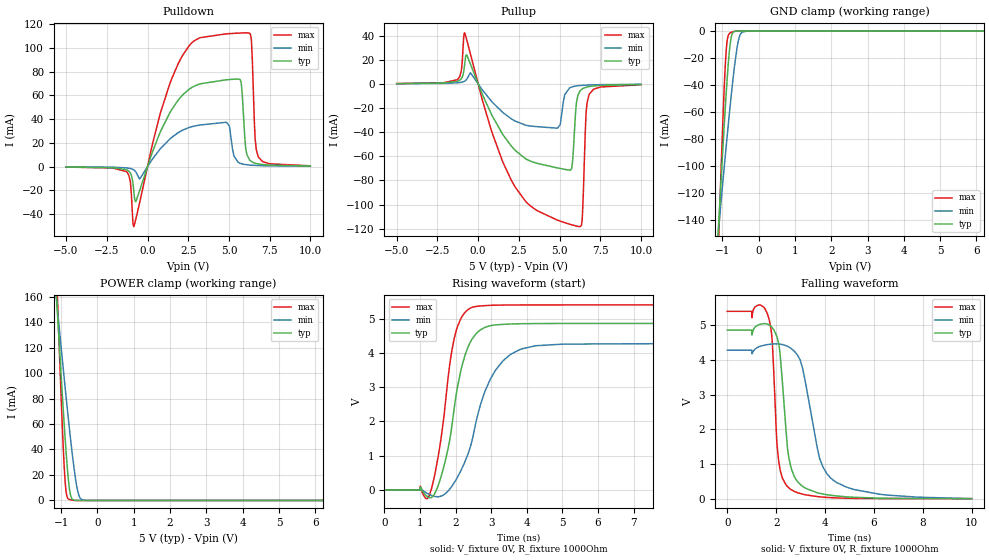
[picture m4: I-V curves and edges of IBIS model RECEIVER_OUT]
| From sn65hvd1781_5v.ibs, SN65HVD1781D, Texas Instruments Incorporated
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|   RECEIVER_OUT Model
[Model]   RECEIVER_OUT
Model_type   Output
| Signals   R
Polarity   Non-Inverting
Enable   Active-High
Vmeas = 2.5
Vref = 2.5
Cref = 15pF
Rref = 1000
| variable   typ   min   max
C_comp   0.74pF   0.68pF   0.82pF
|   typ   min   max
[Voltage Range]   5   4.5   5.5
[Temperature Range]   25   150   -40
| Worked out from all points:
|   slope of the pulldown table from 0 to 0.75 V, typ, clamps not added: 26.6 ohm
|   slope of the pullup table from 0 to 0.75 V, typ, clamps not added: 32.1 ohm
|   GND clamp passes 1 mA (typ) near -0.70 V on its own axis
|   POWER clamp passes 1 mA (typ) near -0.69 V on its own axis
|   falling waveform, V_fixture 0V, R_fixture 1000Ohm: 20-80 % time 387ps typ, 786ps min, 249ps max; typ from 4.86 V to -0.001 V
|   rising waveform, V_fixture 0V, R_fixture 1000Ohm: 20-80 % time 514ps typ, 806ps min, 415ps max; typ from -0.001 V to 4.86 V
[Pulldown]
| Non-monotonic behavior is expected as a consequence of circuit design
|   Voltage   I(typ)   I(min)   I(max)
-5V       -292.3uA   -182.5uA   -355.9uA
-1.295V   -2.615mA   -1.069mA   -4.183mA
-845mV    -20.19mA   -2.707mA   -50.61mA
812.5mV   30.03mA    15.41mA    46.12mA
2.163V    60.52mA    30.8mA     93.99mA
4.855V    73.27mA    37.4mA     112.1mA
5.695V    73.32mA    2.76mA     112.7mA
6.055V    13.33mA    1.64mA     112.9mA
6.362V    4.439mA    1.213mA    108.7mA
6.603V    2.888mA    1.007mA    24.61mA
6.798V    2.245mA    884.5uA    8.31mA
9.992V    476.5uA    293.2uA    664.2uA
[GND Clamp]
| High Current due to TISpice simulations which do not match silicon
| High operating voltage drives high currents.
| Non-monotonic behavior is expected near 0V with small currents.
|   Voltage   I(typ)   I(min)   I(max)
-5V       -2.27A     -1.411A    -3.663A
-1.107V   -146mA     -147.8mA   -160.6mA
-1.093V   -138.6mA   -143.4mA   -148.6mA
-987.5mV  -88.11mA   -112.4mA   -68.55mA
-905mV    -51.15mA   -88.69mA   -19.27mA
-860mV    -33.03mA   -76.05mA   -5.989mA
-807.5mV  -15.47mA   -61.68mA   -1.94mA
-725mV    -1.911mA   -40.27mA   -630.7uA
-597.5mV  -18.86uA   -12.9mA    -19.83uA
-537.5mV  18.77uA    -4.964mA   15.69uA
-297.5mV  25.6uA     9.488uA    22.75uA
10V       0A         0A         0A
[Pullup]
| Non-monotonic behavior is expected as a consequence of circuit design
|   Voltage   I(typ)   I(min)   I(max)
-5V       237.8uA    159.5uA    297uA
-1.272V   2.134mA    940.4uA    3.534mA
-830mV    15.71mA    2.327mA    42.37mA
1.48V     -41.14mA   -23.24mA   -63.45mA
3.603V    -65.74mA   -35.4mA    -104.9mA
4.878V    -69.66mA   -36.65mA   -112.9mA
5.74V     -70.05mA   -2.558mA   -116.7mA
6.228V    -6.335mA   -1.361mA   -118.2mA
6.385V    -4.201mA   -1.18mA    -112.6mA
6.617V    -2.792mA   -986.1uA   -26.69mA
6.812V    -2.175mA   -866.1uA   -8.845mA
9.992V    -466.5uA   -288.1uA   -706.7uA
[POWER Clamp]
| High Current due to TISpice simulations which do not match silicon
| High operating voltage drives high currents.
| Non-monotonic behavior is expected near 0V with small currents.
|   Voltage   I(typ)   I(min)   I(max)
-5V       2.196A     1.366A     3.571A
-1.145V   168.8mA    163.2mA    195.2mA
-1.107V   150.4mA    152.1mA    164.9mA
-1.062V   128.5mA    138.8mA    129.3mA
-957.5mV  79.02mA    108.3mA    52.42mA
-905mV    55.77mA    93.32mA    21.99mA
-852.5mV  34.41mA    78.6mA     5.106mA
-770mV    9.097mA    56.23mA    737.6uA
-710mV    1.726mA    40.85mA    328.1uA
-582.5mV  2.675uA    13.32mA    -22.1uA
-432.5mV  -35.01uA   623.9uA    -32.11uA
10V       0A         0A         0A
[Ramp]
R_load = 1000
|   typ   min   max
dV/dt_r   2.91552/5.13373e-10   2.56841/8.05708e-10   3.23934/4.1332e-10
dV/dt_f   2.91552/3.86492e-10   2.56841/7.79766e-10   3.23934/2.48182e-10
[Falling Waveform]
V_fixture = 0V
V_fixture_min = 0V
V_fixture_max = 0V
R_fixture = 1000Ohm
C_fixture = 0F
|   Time   V(typ)   V(min)   V(max)
0s        4.858V     4.278V     5.398V
1.65ns    5.029V     4.44V      5.313V
1.835ns   4.931V     4.455V     4.587V
2.02ns    4.686V     4.459V     1.736V
2.1ns     4.482V     4.456V     1.112V
2.57ns    1.007V     4.348V     280.5mV
2.985ns   411.3mV    3.994V     146.4mV
3.765ns   154.8mV    1.197V     52.63mV
4.245ns   95.59mV    582.3mV    27.55mV
9.995ns   -1.093mV   -2.325mV   -690.9uV
[Rising Waveform]
V_fixture = 0V
V_fixture_min = 0V
V_fixture_max = 0V
R_fixture = 1000Ohm
C_fixture = 0F
|   Time   V(typ)   V(min)   V(max)
0s        -1.093mV   -2.325mV   -690.9uV
1.01ns    87.02mV    64.37mV    109.5mV
1.25ns    -224.5mV   -128mV     -190.3mV
1.6ns     418.6mV    -179mV     1.571V
1.955ns   2.341V     200.5mV    4.391V
2.155ns   3.516V     577.5mV    5.014V
2.415ns   4.315V     1.262V     5.305V
2.965ns   4.791V     3.206V     5.386V
3.785ns   4.848V     4.086V     5.397V
9.995ns   4.858V     4.278V     5.398V
